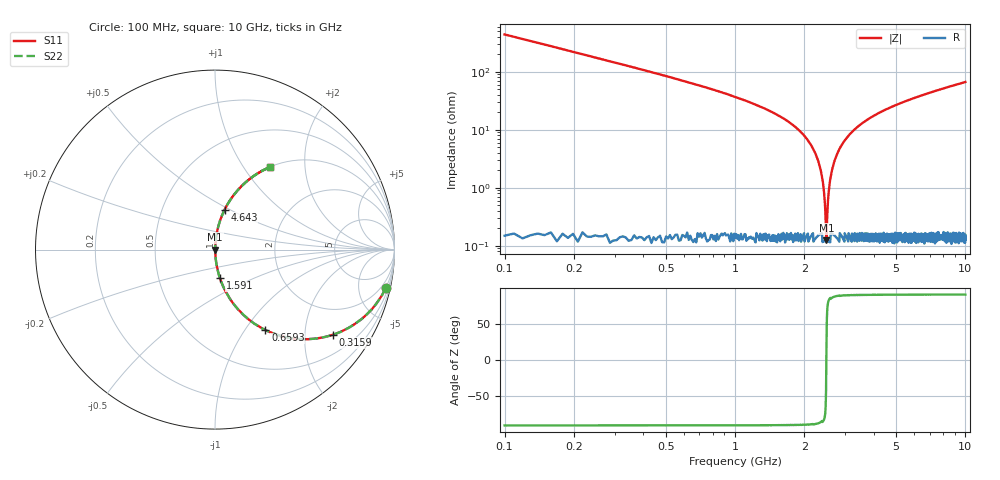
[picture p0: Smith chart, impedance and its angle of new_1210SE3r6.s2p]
!	AVX	Thin	Film	Operation	Date:	April 2007
!	Description:	Accu-P®	"Series,"	Thin	"Film,"	"SMD,"	RF	Capacitor
!	Part	Number:	12101J0R6ABT
!	100	MHz	-	6.05	GHz
!	Serial	Measurements
#	MHZ	S	MA	R	50
!	S11	S21	S12	S22
!	dB	Phase	dB	Phase	dB	Phase	dB	Phase
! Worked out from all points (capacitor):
!   1010 points, 100 MHz to 10 GHz, reference 50 ohm
!   read as one part in series: C = 3.6 pF near 149.1 MHz
!   lowest |Z| = 124 mohm at 2.494 GHz (marker M1)
!   series resonance near 2.492 GHz, so ESL is about 1.1 nH
!   S11 on the Smith chart (normalised r, x): 100 MHz: 1.01, -8.83; 315.9 MHz: 1.00, -2.76; 659.3 MHz: 1.00, -1.25; 1.591 GHz: 1.00, -0.33; 4.643 GHz: 1.00, +0.47; 10 GHz: 1.00, +1.34
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100  0.975 -12.8  0.221 77.2  0.221 77.2  0.975 -12.8
315.857  0.809 -36.0  0.587 54.0  0.587 54.0  0.809 -36.0
659.267  0.529 -58.0  0.848 31.9  0.848 31.9  0.529 -58.0
1032.111  0.334 -70.3  0.941 19.5  0.941 19.5  0.334 -70.3
1591.378  0.162 -80.2  0.985 9.3  0.985 9.3  0.162 -80.2
1758.176  0.125 -82.2  0.991 7.2  0.991 7.2  0.125 -82.2
2062.339  0.067 -85.0  0.996 3.9  0.996 3.9  0.067 -85.0
2268.385  0.033 -85.7  0.998 1.9  0.998 1.9  0.033 -85.7
2376.313  0.017 -84.3  0.998 1.0  0.998 1.0  0.017 -84.3
2454.807  0.00549 -74.9  0.999 0.3  0.999 0.3  0.00549 -74.9
2494.054  0.00143 12.8  0.999 -0.0  0.999 -0.0  0.00143 12.8
2523.489  0.00469 72.4  0.999 -0.3  0.999 -0.3  0.00469 72.4
2572.547  0.011 82.3  0.999 -0.6  0.999 -0.6  0.011 82.3
2611.794  0.017 84.2  0.998 -1.0  0.998 -1.0  0.017 84.2
2758.969  0.036 85.7  0.998 -2.1  0.998 -2.1  0.036 85.7
3004.262  0.067 85.0  0.996 -3.8  0.996 -3.8  0.067 85.0
3406.541  0.112 82.9  0.992 -6.4  0.992 -6.4  0.112 82.9
4642.815  0.229 76.4  0.972 -13.2  0.972 -13.2  0.229 76.4
5054.906  0.263 74.5  0.964 -15.2  0.964 -15.2  0.263 74.5
6703.271  0.38 67.5  0.924 -22.3  0.924 -22.3  0.38 67.5
8351.635  0.476 61.4  0.878 -28.4  0.878 -28.4  0.476 61.4
10000  0.555 56.2  0.831 -33.7  0.831 -33.7  0.555 56.2
